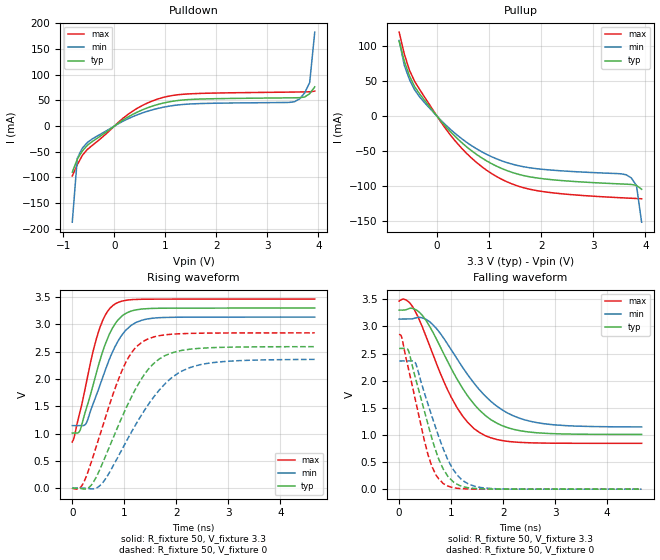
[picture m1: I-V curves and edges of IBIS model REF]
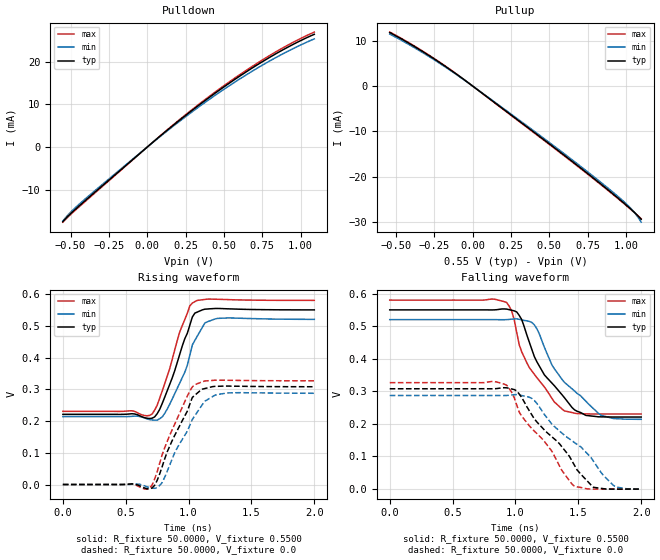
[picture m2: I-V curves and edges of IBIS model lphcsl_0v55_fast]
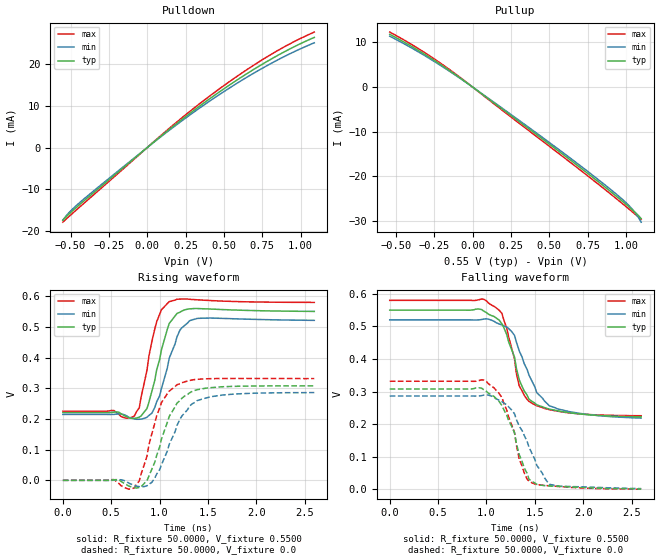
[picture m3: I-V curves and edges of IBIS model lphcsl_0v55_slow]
| Integrated Devices Technolgy, Inc
[IBIS Ver]   4.1
[File name]   9fgl0841.ibs
[File Rev]   1.0
|Rev history   1.0   original ibis data
[Date]   12 October, 2015
[Disclaimer] Integrated Device Technology, Inc. ("IDT") hereby grants the
   user of this ibis model a non-exclusive, nontransferable
   license to use this ibis model under the following terms. the
   user is granted this license only to use the ibis model and is
   not granted rights to sell, copy (except as needed to run the
   ibis model), rent, lease or sub-license the ibis model in
   whole or in part, or in modified form to anyone. the user may
   modify the ibis model to suit its specific applications, but
   rights to derivative works and such modifications shall belong
   to idt. this ibis model is provided on an as is" basis and idt
   makes absolutely no warranty with respect to the information
   contained herein. idt disclaims and customer waives all
   warranties, express and implied, including warranties of
   merchantability and fitness for a particular purpose. the
   entire risk as to quality and performance is with the user
   accordingly, in no event shall idt be liable for any direct or
   indirect damages, whether in contract or tort, including any
   lost profits or other incidental, consequential, exemplary, or
   punitive damages arising out of the use or application of the
   ibis model. further, idt reserves the right to make changes
   without notice to any product herein to improve reliability,
   function, or design. idt does not convey any license under
   patent rights or any other intellectual property rights,
   including those of third parties. idt is not obligated to
   provide maintenance or support for the licensed ibis model.
[Copyright]   Copyright 2012, Integrated Devices Technolgy, Inc. all rights
   reserved
[Component]   9fgl0841
[Manufacturer] Integrated Device Technology, Inc.
[Package]
R_pkg   72.4655m   58.886m   86.045m
L_pkg   1.47175nH   1.11650nH   1.77850nH
C_pkg   0.07747pF   0.07444pF   0.08050pF
[Pin] signal_name  model_name
1   vSS_EN_tri   GND
2   GNDXTAL   GND
3   XIN/CLKIN_25   X1
4   X2   X2
5   VDDXTAL3.3   POWER
6   VDDREF3.3   POWER
7   vSADR/REF3.3   REF
8   GNDREF   GND
9   GNDDIG   GND
10   SCLK_3.3   SCIN
11   SDATA_3.3   SCIN
12   VDDDIG3.3   POWER
13   VDDIO   POWER
14   vOE0#   IN
15   DIF0   LP_HCSL
16   DIF0#   LP_HCSL
17   vOE1#   IN
18   DIF1   LP_HCSL
19   DIF1#   LP_HCSL
20   VDD3.3   POWER
21   VDDIO   POWER
22   GND   GND
23   DIF2   LP_HCSL
24   DIF2#   LP_HCSL
25   vOE2#   IN
26   DIF3   LP_HCSL
27   DIF3#   LP_HCSL
28   vOE3#   IN
29   GNDA   GND
30   VDDA3.3   POWER
31   VDDIO   POWER
32   DIF4   LP_HCSL
33   DIF4#   LP_HCSL
34   vOE4#   IN
35   DIF5   LP_HCSL
36   DIF5#   LP_HCSL
37   vOE5#   IN
38   VDD3.3   POWER
39   VDDIO   POWER
40   GND   GND
41   DIF6   LP_HCSL
42   DIF6#   LP_HCSL
43   vOE6#   IN
44   DIF7   LP_HCSL
45   DIF7#   LP_HCSL
46   vOE7#   IN
47   VDDIO   POWER
48   ^CKPWRGD_PD#   PD
49   ePAD   GND
[Diff Pin]  inv_pin  vdiff tdelay_typ tdelay_min  tdelay_max
15   16   NA   0   0   0
18   19   NA   0   0   0
23   24   NA   0   0   0
26   27   NA   0   0   0
32   33   NA   0   0   0
35   36   NA   0   0   0
41   42   NA   0   0   0
44   45   NA   0   0   0
[Model Selector] LP_HCSL
lphcsl_0v55_fast amplitude 0.55V, slew rate fast
lphcsl_0v55_slow amplitude 0.55V, slew rate slow
lphcsl_0v65_fast amplitude 0.65V, slew rate fast
lphcsl_0v65_slow amplitude 0.65V, slew rate slow
lphcsl_0v7_fast amplitude 0.7V, slew rate fast
lphcsl_0v7_slow amplitude 0.7V, slew rate slow
lphcsl_0v8_fast amplitude 0.8V, slew rate fast
lphcsl_0v8_slow amplitude 0.8V, slew rate slow
| Models and submodels in the file (14): REF (Output), lphcsl_0v55_fast (Output), lphcsl_0v55_slow (Output), lphcsl_0v65_fast (Output), lphcsl_0v65_slow (Output), lphcsl_0v7_fast (Output), lphcsl_0v7_slow (Output), lphcsl_0v8_fast (Output), lphcsl_0v8_slow (Output), SCIN (Input), IN (Input), PD (Input), X1 (Input), X2 (Output)
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[Model]   REF
Model_type   Output
Polarity   Non-Inverting
|   typ   min   max
C_comp   2pF   1.5pF   2.5pF
Vmeas = 1.65V
Rref = 50
Cref = 0
Vref = 1.65V
|   typ   min   max
[Voltage range]   3.3V   3.135V   3.465V
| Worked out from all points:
|   slope of the pulldown table from 0 to 0.495 V, typ, clamps not added: 16.9 ohm
|   slope of the pullup table from 0 to 0.495 V, typ, clamps not added: 12.6 ohm
|   rising waveform, R_fixture 50, V_fixture 3.3: 20-80 % time 450ps typ, 507ps min, 388ps max; typ from 1.01 V to 3.3 V
|   falling waveform, R_fixture 50, V_fixture 3.3: 20-80 % time 857ps typ, 970ps min, 739ps max; typ from 3.3 V to 1.01 V
|   rising waveform, R_fixture 50, V_fixture 0: 20-80 % time 771ps typ, 936ps min, 618ps max; typ from 0 V to 2.59 V
|   falling waveform, R_fixture 50, V_fixture 0: 20-80 % time 472ps typ, 527ps min, 413ps max; typ from 2.59 V to 0 V
[Pulldown]
|Voltage   I (typ)   I (min)   I (max)
|Note, modeling breaks down at 250mA and above.  This is well beyond the functional   |
|operating range of the device.  Should this scenario occur, catastrophic failure and   |
|possible damage to the device and/or board is of higher concern than the I-V curve   |
|behavior.  The IBIS checker will flag currents in excess of 10A with warnings.  Lines   |
|with currents in excess of 0.35 A have been commented out.  The points still remain|
|available to the user if the user desires to use them.   |
|-3.30000e+00   -4.58626e+02   -3.98855e+02   -5.58913e+02
|-3.20100e+00   -4.38670e+02   -3.81813e+02   -5.34126e+02
|-3.10200e+00   -4.18718e+02   -3.64776e+02   -5.09343e+02
|-3.00300e+00   -3.98770e+02   -3.47745e+02   -4.84563e+02
|-2.90400e+00   -3.78827e+02   -3.30720e+02   -4.59787e+02
|-2.80500e+00   -3.58890e+02   -3.13701e+02   -4.35015e+02
|-2.70600e+00   -3.38959e+02   -2.96690e+02   -4.10248e+02
|-2.60700e+00   -3.19035e+02   -2.79688e+02   -3.85486e+02
|-2.50800e+00   -2.99119e+02   -2.62696e+02   -3.60731e+02
|-2.40900e+00   -2.79213e+02   -2.45715e+02   -3.35984e+02
|-2.31000e+00   -2.59319e+02   -2.28747e+02   -3.11245e+02
|-2.21100e+00   -2.39437e+02   -2.11796e+02   -2.86516e+02
|-2.11200e+00   -2.19572e+02   -1.94864e+02   -2.61800e+02
|-2.01300e+00   -1.99726e+02   -1.77955e+02   -2.37100e+02
|-1.91400e+00   -1.79905e+02   -1.61075e+02   -2.12419e+02
|-1.81500e+00   -1.60116e+02   -1.44233e+02   -1.87763e+02
|-1.71600e+00   -1.40369e+02   -1.27441e+02   -1.63140e+02
|-1.61700e+00   -1.20682e+02   -1.10717e+02   -1.38565e+02
|-1.51800e+00   -1.01080e+02   -9.40899e+01   -1.14061e+02
|-1.41900e+00   -8.16135e+01   -7.76121e+01   -8.96701e+01
|-1.32000e+00   -6.23864e+01   -6.13830e+01   -6.54941e+01
|-1.22100e+00   -4.36066e+01   -4.55730e+01   -4.17841e+01
|-1.12200e+00   -2.55446e+01   -3.03740e+01   -1.89497e+01
|-1.02300e+00   -8.13369e+00   -1.57511e+01   -1.01906e+00
|-9.24000e-01   -3.55892e-01   -2.38948e+00   -1.27879e-01
-825mV    -89.74mA   -186.9mA   -97.05mA
-726mV    -64.34mA   -62.46mA   -75.03mA
-627mV    -48.3mA    -42.65mA   -56.86mA
-528mV    -37.22mA   -31.89mA   -45.33mA
363mV     22.88mA    18.45mA    29.33mA
957mV     44.74mA    36.62mA    55.73mA
1.551V    52.05mA    43.3mA     63.04mA
3.531V    55.03mA    47.39mA    66.19mA
3.63V     55.21mA    52.95mA    66.32mA
3.729V    56.59mA    64.36mA    66.46mA
3.828V    63.02mA    84.81mA    66.64mA
3.927V    76.26mA    182.8mA    67.99mA
| 4.02600e+00   9.63336e-02   1.95544e+00   7.56685e-02
| 4.12500e+00   1.29319e-01   1.96109e+01   9.19025e-02
| 4.22400e+00   6.62462e-01   4.21550e+01   1.15435e-01
| 4.32300e+00   1.51637e+01   6.47670e+01   1.37492e-01
| 4.42200e+00   4.22442e+01   8.74545e+01   2.35006e-01
| 4.52100e+00   6.94172e+01   1.10195e+02   8.92943e+00
| 4.62000e+00   9.66780e+01   1.32968e+02   4.35589e+01
| 4.71900e+00   1.23991e+02   1.55761e+02   7.83218e+01
| 4.81800e+00   1.51333e+02   1.78569e+02   1.13180e+02
| 4.91700e+00   1.78693e+02   2.01386e+02   1.48085e+02
| 5.01600e+00   2.06065e+02   2.24210e+02   1.83014e+02
| 5.11500e+00   2.33446e+02   2.47041e+02   2.17958e+02
| 5.21400e+00   2.60834e+02   2.69877e+02   2.52912e+02
| 5.31300e+00   2.88228e+02   2.92717e+02   2.87874e+02
| 5.41200e+00   3.15625e+02   3.15560e+02   3.22841e+02
| 5.51100e+00   3.43027e+02   3.38407e+02   3.57813e+02
| 5.61000e+00   3.70432e+02   3.61256e+02   3.92789e+02
| 5.70900e+00   3.97841e+02   3.84108e+02   4.27769e+02
| 5.80800e+00   4.25252e+02   4.06963e+02   4.62752e+02
| 5.90700e+00   4.52666e+02   4.29821e+02   4.97738e+02
| 6.00600e+00   4.80082e+02   4.52680e+02   5.32727e+02
| 6.10500e+00   5.07501e+02   4.75543e+02   5.67718e+02
| 6.20400e+00   5.34922e+02   4.98407e+02   6.02711e+02
| 6.30300e+00   5.62345e+02   5.21273e+02   6.37705e+02
| 6.40200e+00   5.89770e+02   5.44142e+02   6.72701e+02
| 6.50100e+00   6.17197e+02   5.67013e+02   7.07699e+02
| 6.60000e+00   6.44626e+02   5.89886e+02   7.42698e+02
[Pullup]
|Voltage   I (typ)   I (min)   I (max)
|Note, modeling breaks down at 250mA and above.  This is well beyond the functional   |
|operating range of the device.  Should this scenario occur, catastrophic failure and   |
|possible damage to the device and/or board is of higher concern than the I-V curve   |
|behavior.  The IBIS checker will flag currents in excess of 10A with warnings.  Lines   |
|with currents in excess of 0.35 A have been commented out.  The points still remain|
|available to the user if the user desires to use them.   |
|-3.30000e+00   6.44680e+02   5.51825e+02   8.01095e+02
|-3.20100e+00   6.17254e+02   5.28958e+02   7.66095e+02
|-3.10200e+00   5.89830e+02   5.06093e+02   7.31096e+02
|-3.00300e+00   5.62407e+02   4.83230e+02   6.96098e+02
|-2.90400e+00   5.34987e+02   4.60368e+02   6.61102e+02
|-2.80500e+00   5.07568e+02   4.37509e+02   6.26108e+02
|-2.70600e+00   4.80150e+02   4.14651e+02   5.91115e+02
|-2.60700e+00   4.52735e+02   3.91796e+02   5.56124e+02
|-2.50800e+00   4.25322e+02   3.68942e+02   5.21136e+02
|-2.40900e+00   3.97911e+02   3.46091e+02   4.86149e+02
|-2.31000e+00   3.70503e+02   3.23243e+02   4.51165e+02
|-2.21100e+00   3.43097e+02   3.00397e+02   4.16183e+02
|-2.11200e+00   3.15694e+02   2.77554e+02   3.81204e+02
|-2.01300e+00   2.88295e+02   2.54715e+02   3.46229e+02
|-1.91400e+00   2.60900e+02   2.31881e+02   3.11257e+02
|-1.81500e+00   2.33510e+02   2.09052e+02   2.76290e+02
|-1.71600e+00   2.06127e+02   1.86229e+02   2.41329e+02
|-1.61700e+00   1.78751e+02   1.63415e+02   2.06375e+02
|-1.51800e+00   1.51388e+02   1.40613e+02   1.71432e+02
|-1.41900e+00   1.24042e+02   1.17829e+02   1.36506e+02
|-1.32000e+00   9.67252e+01   9.50724e+01   1.01609e+02
|-1.22100e+00   6.94599e+01   7.23604e+01   6.67700e+01
|-1.12200e+00   4.22820e+01   4.97173e+01   3.20469e+01
|-1.02300e+00   1.51962e+01   2.71494e+01   2.11287e+00
|-9.24000e-01   6.89030e-01   5.34223e+00   1.97623e-01
|-8.25000e-01   1.48916e-01   3.54714e-01   1.54087e-01
-726mV    106.9mA    108.2mA    120.1mA
-627mV    78.63mA    72.64mA    88.74mA
-528mV    57.36mA    52.3mA     65.5mA
-330mV    31.45mA    27.24mA    37.82mA
363mV     -30.02mA   -25.58mA   -36.52mA
957mV     -64.05mA   -54.65mA   -77.43mA
1.353V    -77.99mA   -66.51mA   -94.06mA
1.848V    -87.45mA   -74.38mA   -105.4mA
3.63V     -97.08mA   -83.63mA   -116.9mA
3.729V    -97.47mA   -88.18mA   -117.2mA
3.828V    -98.9mA    -99mA      -117.5mA
3.927V    -104.4mA   -151.4mA   -117.9mA
| 4.02600e+00   -1.15410e-01   -9.65481e-01   -1.19366e-01
| 4.12500e+00   -1.36603e-01   -1.09884e+01   -1.26324e-01
| 4.22400e+00   -3.99361e-01   -2.54841e+01   -1.40663e-01
| 4.32300e+00   -8.17474e+00   -4.04654e+01   -1.58277e-01
| 4.42200e+00   -2.55843e+01   -5.60873e+01   -2.17491e-01
| 4.52100e+00   -4.36450e+01   -7.21990e+01   -4.28595e+00
| 4.62000e+00   -6.24226e+01   -8.86071e+01   -2.64922e+01
| 4.71900e+00   -8.16508e+01   -1.05189e+02   -4.96573e+01
| 4.81800e+00   -1.01115e+02   -1.21884e+02   -7.35635e+01
| 4.91700e+00   -1.20715e+02   -1.38656e+02   -9.78285e+01
| 5.01600e+00   -1.40403e+02   -1.55482e+02   -1.22263e+02
| 5.11500e+00   -1.60149e+02   -1.72350e+02   -1.46794e+02
| 5.21400e+00   -1.79938e+02   -1.89250e+02   -1.71387e+02
| 5.31300e+00   -1.99760e+02   -2.06175e+02   -1.96022e+02
| 5.41200e+00   -2.19606e+02   -2.23121e+02   -2.20688e+02
| 5.51100e+00   -2.39472e+02   -2.40084e+02   -2.45378e+02
| 5.61000e+00   -2.59355e+02   -2.57061e+02   -2.70086e+02
| 5.70900e+00   -2.79251e+02   -2.74051e+02   -2.94808e+02
| 5.80800e+00   -2.99159e+02   -2.91052e+02   -3.19543e+02
| 5.90700e+00   -3.19077e+02   -3.08062e+02   -3.44288e+02
| 6.00600e+00   -3.39003e+02   -3.25080e+02   -3.69042e+02
| 6.10500e+00   -3.58937e+02   -3.42106e+02   -3.93803e+02
| 6.20400e+00   -3.78878e+02   -3.59138e+02   -4.18571e+02
| 6.30300e+00   -3.98826e+02   -3.76177e+02   -4.43346e+02
| 6.40200e+00   -4.18779e+02   -3.93221e+02   -4.68125e+02
| 6.50100e+00   -4.38737e+02   -4.10271e+02   -4.92910e+02
| 6.60000e+00   -4.58699e+02   -4.27325e+02   -5.17700e+02
[Ramp]
|   typ   min   max
dV/dt_r   1.566/0.774n   1.425/0.94n   1.718/0.621n
dV/dt_f   1.396/0.866n   1.212/0.979n   1.595/0.746n
R_load =   50
[Rising Waveform]
R_fixture = 50
V_fixture = 3.3   |Vcc_typ
V_fixture_min = 3.135 |Vcc_min
V_fixture_max = 3.465 |Vcc_max
C_fixture = 0.0p
| Time   typ   min   max
0s        1.008V     1.145V     844.6mV
34.71ps   1.008V     1.145V     923.1mV
154.3ps   1.071V     1.145V     1.413V
275.2ps   1.472V     1.202V     1.956V
479.5ps   2.168V     1.745V     2.789V
635.5ps   2.641V     2.166V     3.174V
823.7ps   3.01V      2.596V     3.375V
1.129ns   3.244V     2.981V     3.453V
1.433ns   3.289V     3.099V     3.463V
4.662ns   3.3V       3.135V     3.465V
[Falling Waveform]
R_fixture = 50
V_fixture = 3.3   |Vcc_typ
V_fixture_min = 3.135 |Vcc_min
V_fixture_max = 3.465 |Vcc_max
C_fixture = 0.0p
| Time   typ   min   max
0s        3.3V       3.135V     3.465V
120.3ps   3.304V     3.135V     3.493V
247.8ps   3.333V     3.138V     3.377V
425ps     3.225V     3.162V     3.038V
624.4ps   2.937V     3.054V     2.545V
1.111ns   2.034V     2.407V     1.506V
1.539ns   1.462V     1.838V     1.048V
1.979ns   1.171V     1.463V     896.3mV
2.515ns   1.052V     1.252V     854.4mV
4.666ns   1.008V     1.146V     844.6mV
[Rising Waveform]
R_fixture = 50
V_fixture = 0
C_fixture = 0.0p
| Time   typ   min   max
0s        23.89nV    60.43nV    30.4nV
191.1ps   -13.44mV   129.7uV    54.48mV
415.8ps   124mV      -13.01mV   625.4mV
623.1ps   548.9mV    147.1mV    1.254V
939.4ps   1.267V     680mV      2.117V
1.156ns   1.708V     1.059V     2.505V
1.348ns   2.027V     1.367V     2.681V
1.787ns   2.43V      1.916V     2.809V
2.339ns   2.554V     2.232V     2.838V
4.662ns   2.593V     2.359V     2.845V
[Falling Waveform]
R_fixture = 50
V_fixture = 0
C_fixture = 0.0p
| Time   typ   min   max
0s        2.593V     2.362V     2.845V
47.92ps   2.593V     2.362V     2.804V
169.8ps   2.571V     2.362V     2.258V
309ps     2.063V     2.332V     1.656V
482.9ps   1.445V     1.783V     905.2mV
624.2ps   958.6mV    1.36V      434.3mV
847.8ps   371.4mV    743.3mV    103.8mV
1.113ns   93.12mV    264.4mV    16.96mV
1.53ns    8.102mV    37.41mV    1.012mV
4.662ns   -1.039uV   -794nV     -867.7nV
[Model]   lphcsl_0v55_fast
Model_type Output
Polarity   Non-Inverting
Enable   Active-High
Vmeas =  0.4000V
Cref =   2.0000pF
Rref =   0.0
Vref =   0.4000V
C_comp   1.1000pF   1.0000pF   1.2000pF
[Temperature Range]   25.0000   85.0000   -40.0
[Voltage Range]   0.5500V   0.5200V   0.5800V
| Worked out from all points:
|   slope of the pulldown table from 0 to 0.083 V, typ, clamps not added: 32.7 ohm
|   slope of the pullup table from 0 to 0.083 V, typ, clamps not added: 39.3 ohm
|   rising waveform, R_fixture 50.0000, V_fixture 0.5500: 20-80 % time 174ps typ, 180ps min, 165ps max; typ from 0.221 V to 0.55 V
|   rising waveform, R_fixture 50.0000, V_fixture 0.0: 20-80 % time 210ps typ, 226ps min, 201ps max; typ from 0 V to 0.308 V
|   falling waveform, R_fixture 50.0000, V_fixture 0.5500: 20-80 % time 295ps typ, 339ps min, 258ps max; typ from 0.55 V to 0.221 V
|   falling waveform, R_fixture 50.0000, V_fixture 0.0: 20-80 % time 385ps typ, 441ps min, 351ps max; typ from 0.308 V to 0 V
[Pulldown]
|Voltage   I(typ)   I(min)   I(max)
-550mV    -17.42mA   -17.31mA   -17.56mA
-510mV    -15.92mA   -15.61mA   -16.12mA
-470mV    -14.59mA   -14.21mA   -14.8mA
-310mV    -9.584mA   -9.264mA   -9.753mA
90mV      2.747mA    2.637mA    2.806mA
350mV     10.16mA    9.756mA    10.37mA
570mV     15.8mA     15.17mA    16.12mA
750mV     19.95mA    19.15mA    20.36mA
910mV     23.24mA    22.29mA    23.72mA
1.09V     26.39mA    25.32mA    26.91mA
[Pullup]
|Voltage   I(typ)   I(min)   I(max)
-540mV    11.78mA    11.45mA    11.88mA
-360mV    8.313mA    8.057mA    8.417mA
-160mV    3.912mA    3.778mA    3.974mA
0V        -107.6pA   -683pA     -85.53pA
480mV     -12.23mA   -11.94mA   -12.36mA
760mV     -19.55mA   -19.19mA   -19.69mA
960mV     -25.05mA   -24.7mA    -25.17mA
1.04V     -27.39mA   -27.28mA   -27.47mA
1.08V     -28.69mA   -28.98mA   -28.66mA
1.1V      -29.42mA   -30.05mA   -29.29mA
[Ramp]
| variable   typ   min   max
dV/dt_r  0.1848/0.2165n   0.1724/0.2461n   0.1960/0.2011n
dV/dt_f  0.1973/0.2848n   0.1835/0.3291n   0.2098/0.2758n
R_load = 50.0000
[Rising Waveform]
R_fixture= 50.0000
V_fixture= 0.5500
V_fixture_min= 0.5200
V_fixture_max= 0.5800
|time   V(typ)   V(min)   V(max)
0s        221mV      213.9mV    230.4mV
710ps     208.9mV    203.3mV    222mV
770ps     236.5mV    207.1mV    271.8mV
830ps     295.1mV    237.4mV    341.4mV
930ps     410.6mV    320mV      481.3mV
1.01ns    502mV      407.6mV    562.8mV
1.07ns    543.3mV    467.9mV    580.1mV
1.13ns    552.4mV    509.1mV    583mV
1.23ns    554.6mV    523.3mV    583.5mV
2ns       550.1mV    520.2mV    580mV
[Rising Waveform]
R_fixture= 50.0000
V_fixture= 0.0
V_fixture_min= 0.0
V_fixture_max= 0.0
|time   V(typ)   V(min)   V(max)
0s        0V         0V         0V
690ps     -13.76mV   -9.908mV   -11mV
730ps     -2.555mV   -12mV      17.28mV
790ps     56.31mV    6.206mV    93.42mV
890ps     155mV      100.6mV    190.4mV
990ps     231mV      167.8mV    278.9mV
1.05ns    281.3mV    216.8mV    314.6mV
1.13ns    302.4mV    262.5mV    326.1mV
1.23ns    309.3mV    283.7mV    328.7mV
2ns       308mV      287.4mV    326.7mV
[Falling Waveform]
R_fixture= 50.0000
V_fixture= 0.5500
V_fixture_min= 0.5200
V_fixture_max= 0.5800
|time   V(typ)   V(min)   V(max)
0s        550mV      520mV      580mV
930ps     552.4mV    520.1mV    572.5mV
970ps     548.8mV    521.6mV    546.6mV
1.03ns    533mV      521mV      442.9mV
1.11ns    451.2mV    514.7mV    373mV
1.23ns    350.6mV    435.4mV    313.4mV
1.31ns    317mV      368.9mV    267.2mV
1.47ns    243.2mV    301.1mV    233mV
1.68ns    221.7mV    226.8mV    230.4mV
2ns       221.1mV    214.1mV    230.4mV
[Falling Waveform]
R_fixture= 50.0000
V_fixture= 0.0
V_fixture_min= 0.0
V_fixture_max= 0.0
|time   V(typ)   V(min)   V(max)
0s        307.9mV    287.3mV    326.7mV
890ps     310.7mV    287.1mV    324.6mV
950ps     309.3mV    287.8mV    308.9mV
1.01ns    301.5mV    290mV      257.9mV
1.11ns    240.4mV    281.8mV    194.3mV
1.29ns    160.4mV    199.1mV    116.1mV
1.47ns    72.59mV    142.7mV    8.438mV
1.62ns    5.493mV    86.02mV    77.42uV
1.78ns    -65.96uV   11.35mV    -85.75uV
2ns       -77.45uV   -198.5uV   -34.61uV
[Model]   lphcsl_0v55_slow
Model_type Output
Polarity   Non-Inverting
Enable   Active-High
Vmeas =  0.4000V
Cref =   2.0000pF
Rref =   0.0
Vref =   0.4000V
C_comp   1.1000pF   1.0000pF   1.2000pF
[Temperature Range]   25.0000   85.0000   -40.0000
[Voltage Range]   0.5500V   0.5200V   0.5800V
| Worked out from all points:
|   slope of the pulldown table from 0 to 0.083 V, typ, clamps not added: 32.7 ohm
|   slope of the pullup table from 0 to 0.083 V, typ, clamps not added: 39.3 ohm
|   rising waveform, R_fixture 50.0000, V_fixture 0.5500: 20-80 % time 156ps typ, 172ps min, 137ps max; typ from 0.221 V to 0.551 V
|   rising waveform, R_fixture 50.0000, V_fixture 0.0: 20-80 % time 218ps typ, 257ps min, 187ps max; typ from 0 V to 0.308 V
|   falling waveform, R_fixture 50.0000, V_fixture 0.5500: 20-80 % time 226ps typ, 279ps min, 186ps max; typ from 0.55 V to 0.222 V
|   falling waveform, R_fixture 50.0000, V_fixture 0.0: 20-80 % time 221ps typ, 262ps min, 196ps max; typ from 0.308 V to 0.001 V
[Pulldown]
|Voltage   I(typ)   I(min)   I(max)
-550mV    -17.42mA   -17.37mA   -17.87mA
-510mV    -15.92mA   -15.58mA   -16.5mA
-470mV    -14.59mA   -14.14mA   -15.2mA
-350mV    -10.82mA   -10.4mA    -11.34mA
70mV      2.144mA    2.042mA    2.274mA
330mV     9.616mA    9.161mA    10.17mA
550mV     15.31mA    14.58mA    16.15mA
730mV     19.51mA    18.57mA    20.56mA
910mV     23.24mA    22.1mA     24.45mA
1.09V     26.39mA    25.1mA     27.67mA
[Pullup]
|Voltage   I(typ)   I(min)   I(max)
-540mV    11.78mA    11.36mA    12.28mA
-360mV    8.313mA    7.995mA    8.73mA
-160mV    3.912mA    3.748mA    4.141mA
40mV      -1.02mA    -975.2uA   -1.083mA
480mV     -12.23mA   -11.87mA   -12.71mA
760mV     -19.55mA   -19.1mA    -20.1mA
960mV     -25.05mA   -24.6mA    -25.58mA
1.04V     -27.39mA   -27.24mA   -27.85mA
1.08V     -28.69mA   -29.05mA   -29.01mA
1.1V      -29.42mA   -30.23mA   -29.61mA
[Ramp]
| variable   typ   min   max
dV/dt_r  0.1848/0.2190n   0.1717/0.2485n   0.1991/0.1882n
dV/dt_f  0.1965/0.2484n   0.1808/0.2865n   0.2125/0.2078n
R_load = 50.0000
[Rising Waveform]
R_fixture= 50.0000
V_fixture= 0.5500
V_fixture_min= 0.5200
V_fixture_max= 0.5800
|time   V(typ)   V(min)   V(max)
0s        221mV      214.9mV    225.3mV
740ps     201.9mV    200.2mV    210mV
790ps     206mV      199.1mV    236.4mV
870ps     234.3mV    205.7mV    359.2mV
920ps     290mV      218.6mV    452mV
1.02ns    426.3mV    299.8mV    556.5mV
1.1ns     511.8mV    398.5mV    582.6mV
1.21ns    548.2mV    489.5mV    591.1mV
1.39ns    560.3mV    528.2mV    588.8mV
2.6ns     550.9mV    521.7mV    580.3mV
[Rising Waveform]
R_fixture= 50.0000
V_fixture= 0.0
V_fixture_min= 0.0
V_fixture_max= 0.0
|time   V(typ)   V(min)   V(max)
0s        0V         0V         0V
550ps     2.324mV    951.5uV    -2.512mV
740ps     -24.18mV   -16.37mV   -24.55mV
790ps     -23.47mV   -20.51mV   -2.409mV
920ps     36.17mV    -6.753mV   151.8mV
1.02ns    135mV      51.17mV    253.8mV
1.18ns    251.8mV    179.1mV    311.9mV
1.31ns    285.3mV    242.2mV    325.5mV
1.52ns    302mV      272.4mV    331.5mV
2.6ns     308mV      286.1mV    331.8mV
[Falling Waveform]
R_fixture= 50.0000
V_fixture= 0.5500
V_fixture_min= 0.5200
V_fixture_max= 0.5800
|time   V(typ)   V(min)   V(max)
0s        550mV      520mV      580mV
970ps     547.5mV    522.6mV    583.6mV
1.16ns    508mV      504.6mV    540.1mV
1.29ns    406.3mV    472.7mV    400.4mV
1.31ns    370.9mV    451.9mV    355.2mV
1.34ns    335.5mV    423.9mV    316.5mV
1.44ns    276.5mV    350.4mV    269.9mV
1.52ns    259.5mV    296.8mV    256.6mV
1.65ns    246.1mV    256.4mV    244.6mV
2.6ns     222.5mV    218.6mV    225.8mV
[Falling Waveform]
R_fixture= 50.0000
V_fixture= 0.0
V_fixture_min= 0.0
V_fixture_max= 0.0
|time   V(typ)   V(min)   V(max)
0s        307.9mV    286.4mV    331.7mV
970ps     306.1mV    289.1mV    335.8mV
1.16ns    257.3mV    269.1mV    282mV
1.29ns    173.9mV    232mV      174.5mV
1.34ns    105.8mV    193.4mV    91.43mV
1.39ns    66.68mV    165.9mV    50.82mV
1.44ns    31.41mV    129mV      24.81mV
1.52ns    15.24mV    73.8mV     14.68mV
1.65ns    10.13mV    15.34mV    10.72mV
2.6ns     993.4uV    2.118mV    402uV
